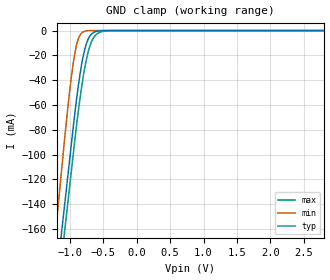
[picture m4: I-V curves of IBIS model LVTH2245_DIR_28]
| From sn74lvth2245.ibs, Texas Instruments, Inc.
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[Model]   LVTH2245_DIR_28
Model_type  Input
Vinl = 0.8
Vinh = 2.0
| variable   typ   min   max
C_comp   4.64pF   3.64pF   5.97pF
[Temperature Range]   40   -40   100
| Ambient temperature   25   -40   85
[Voltage range]   2.8   2.7   2.9
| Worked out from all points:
|   GND clamp passes 1 mA (typ) near -0.62 V on its own axis
[GND Clamp]
| LVTH2245_DIR_28
|   Voltage   I(typ)   I(min)   I(max)
-5.5V     -2.407A    -2.649A    -2.406A
-1.22V    -209.3mA   -166mA     -230mA
-1.205V   -202mA     -157.6mA   -222.8mA
-1.125V   -163.1mA   -113mA     -184.2mA
-1.075V   -138.8mA   -85.25mA   -160.1mA
-975mV    -90.17mA   -36.12mA   -112mA
-900mV    -55.28mA   -11.44mA   -76.47mA
-800mV    -20.27mA   -984.6uA   -36.91mA
-675mV    -2.699mA   -6.758uA   -8.728mA
-575mV    -336.8uA   -57.38nA   -1.991mA
-425mV    -3.297uA   -110.8pA   -102.1uA
2.8V      13.7pA     7.338pA    757.3pA
